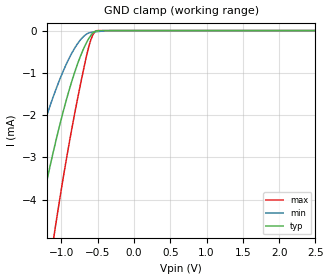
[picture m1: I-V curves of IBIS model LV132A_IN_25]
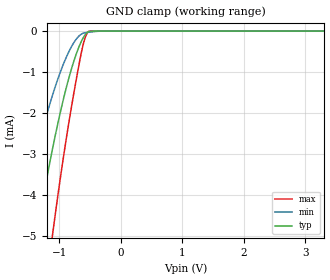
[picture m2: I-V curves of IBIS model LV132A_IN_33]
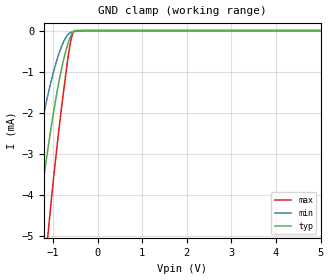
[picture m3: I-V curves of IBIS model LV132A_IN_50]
| TEXAS INSTRUMENTS INCORPORATED
| Standard Linear and Logic Group
| IBIS Model of SN74LV132A
| QUADRUPLE POSITIVE-NAND GATES WITH SCHMITT-TRIGGER INPUTS
| This file contains package information for the following:
|  SOIC 14-pin (D) package as [Component] LV132A_D
|  SSOP 14-pin (DB) package as [Component] LV132A_DB
|  TVSOP 14-pin (DGV) package as [Component] LV132A_DGV
|  SOP 14-pin (NS) package as [Component] LV132A_NS
|  TSSOP 14-pin (PW) package as [Component] LV132A_PW
| This device can be powered at the following Vccs:
|  2.5 volt Vcc
|  3.3 volt Vcc
|  5 volt Vcc
| This file provides unique models under the [Model Selector] for each Vcc.
| For operation at a specific Vcc, select the appropriate model after each
| [Model Selector] keyword.
[IBIS Ver]   3.2
[Comment char]  |_char
[File Name]   sn74lv132a.ibs
[File Rev]   1.1 | h_die
[Date]   February 26, 2004
[Source]   Data created from TI-SPICE simulations at TI-SLL.
[Notes]   The following is an IBIS list for the LV132A.
   Please contact sllibis@ti.com with questions and
   comments concerning SLL IBIS models.
   This IBIS model is created from a BA (back annotated netlist)
   - FILE REV HISTORY
   - 1.1 Release IBIS file on 02/26/04
   - Power clamp data deleted as there is no power-clamp diode.
[Disclaimer] Property of Texas Instruments Incorporated.  Unauthorized
   reproduction and/or distribution is strictly prohibited.
   This product is protected under copyright law.
   Created  2003, (C) Copyright  2003, Texas Instruments
   Incorporated, All Rights Reserved
   UNLESS THERE IS A SIGNED, WRITTEN AGREEMENT TO THE
   CONTRARY, TEXAS INSTRUMENTS (TI) IS PROVIDING THE IBIS
   MODELS  AND WITHOUT ANY WARRANTY, EXPRESSED OR
   IMPLIED.  TI assumes no liability for:
   1) the accuracy of the IBIS models provided to your
   company;
   2) the proper functioning of these IBIS Models in your
   design or for any resulting applications; or
   3) infringement of patents, copyrights or intellectual
   property rights resulting from your use of these IBIS
   models.
   TI provides IBIS Models as a service to our customers.
   You and your company shall not distribute, sell or give
   these models to anyone else without prior written
   permission from TI.
   TI reserves the right to make changes to our products or
   to discontinue any semiconductor product or service
   without notice, and advises our customers to obtain the
   latest version of relevant information to verify, before
   placing orders, that the information being relied on is
   current.
   Please be aware that your receipt and use of the IBIS
   information provided shall serve as acceptance of these
   terms and conditions.  If you do not accept these terms,
   you should return or destroy the IBIS models and any
   other accompanying information immediately.
| Component LV132A_D 14-pin SOIC
[Component]   LV132A_D
[Manufacturer]   Texas Instruments, Inc.
[Package]
|   typ   min   max
R_pkg   3.100e-02   2.800e-02   3.400e-02
L_pkg   3.109e-09   2.462e-09   3.889e-09
C_pkg   4.730e-13   3.630e-13   6.280e-13
[Pin]   signal_name   model_name   R_pin   L_pin   C_pin
1   1A   LV132A_IN   3.300e-02   3.854e-09   6.220e-13
2   1B   LV132A_IN   3.200e-02   3.188e-09   4.730e-13
3   1Y   LV132A_OUT   2.800e-02   2.462e-09   3.770e-13
4   2A   LV132A_IN   3.100e-02   2.596e-09   3.630e-13
5   2B   LV132A_IN   2.800e-02   2.521e-09   3.720e-13
6   2Y   LV132A_OUT   3.400e-02   3.250e-09   4.760e-13
7   GND   GND   3.400e-02   3.889e-09   6.280e-13
8   3Y   LV132A_OUT   3.400e-02   3.889e-09   6.280e-13
9   3A   LV132A_IN   3.400e-02   3.250e-09   4.760e-13
10   3B   LV132A_IN   2.800e-02   2.521e-09   3.720e-13
11   4Y   LV132A_OUT   3.100e-02   2.596e-09   3.640e-13
12   4A   LV132A_IN   2.800e-02   2.462e-09   3.770e-13
13   4B   LV132A_IN   3.200e-02   3.188e-09   4.730e-13
14   VCC   POWER   3.300e-02   3.854e-09   6.220e-13
| Component LV132A_DB 14-pin SSOP
[Component]   LV132A_DB
[Manufacturer]   Texas Instruments, Inc.
[Package]
|   typ   min   max
R_pkg   4.400e-02   4.100e-02   4.600e-02
L_pkg   3.551e-09   3.258e-09   3.927e-09
C_pkg   4.020e-13   3.600e-13   4.210e-13
[Pin]   signal_name   model_name   R_pin   L_pin   C_pin
1   1A   LV132A_IN   4.600e-02   3.927e-09   4.080e-13
2   1B   LV132A_IN   4.400e-02   3.587e-09   4.210e-13
3   1Y   LV132A_OUT   4.100e-02   3.289e-09   3.980e-13
4   2A   LV132A_IN   4.200e-02   3.258e-09   3.600e-13
5   2B   LV132A_IN   4.100e-02   3.286e-09   4.030e-13
6   2Y   LV132A_OUT   4.400e-02   3.586e-09   4.210e-13
7   GND   GND   4.600e-02   3.927e-09   4.080e-13
8   3Y   LV132A_OUT   4.600e-02   3.927e-09   4.080e-13
9   3A   LV132A_IN   4.400e-02   3.586e-09   4.210e-13
10   3B   LV132A_IN   4.100e-02   3.286e-09   4.030e-13
11   4Y   LV132A_OUT   4.300e-02   3.258e-09   3.600e-13
12   4A   LV132A_IN   4.100e-02   3.289e-09   3.980e-13
13   4B   LV132A_IN   4.400e-02   3.587e-09   4.210e-13
14   VCC   POWER   4.600e-02   3.927e-09   4.080e-13
| Component LV132A_DGV 14-pin TVSOP
[Component]   LV132A_DGV
[Manufacturer]   Texas Instruments, Inc.
[Package]
|   typ   min   max
R_pkg   3.500e-02   2.000e-02   4.500e-02
L_pkg   2.499e-09   2.077e-09   2.966e-09
C_pkg   3.610e-13   3.050e-13   4.160e-13
[Pin]   signal_name   model_name   R_pin   L_pin   C_pin
1   1A   LV132A_IN   2.700e-02   2.717e-09   3.730e-13
2   1B   LV132A_IN   3.700e-02   2.434e-09   3.980e-13
3   1Y   LV132A_OUT   3.400e-02   2.200e-09   3.160e-13
4   2A   LV132A_IN   2.000e-02   2.077e-09   3.090e-13
5   2B   LV132A_IN   3.000e-02   2.147e-09   3.050e-13
6   2Y   LV132A_OUT   4.200e-02   2.580e-09   4.080e-13
7   GND   GND   3.900e-02   2.921e-09   3.850e-13
8   3Y   LV132A_OUT   3.300e-02   2.841e-09   3.800e-13
9   3A   LV132A_IN   4.200e-02   2.611e-09   4.100e-13
10   3B   LV132A_IN   3.800e-02   2.331e-09   3.290e-13
11   4Y   LV132A_OUT   2.600e-02   2.223e-09   3.190e-13
12   4A   LV132A_IN   3.400e-02   2.259e-09   3.130e-13
13   4B   LV132A_IN   4.500e-02   2.681e-09   4.160e-13
14   VCC   POWER   4.200e-02   2.966e-09   3.860e-13
| Component LV132A_NS 14-pin SOP
[Component]   LV132A_NS
[Manufacturer]   Texas Instruments, Inc.
[Package]
|   typ   min   max
R_pkg   4.500e-02   3.900e-02   5.400e-02
L_pkg   3.796e-09   2.561e-09   4.952e-09
C_pkg   5.280e-13   2.880e-13   7.100e-13
[Pin]   signal_name   model_name   R_pin   L_pin   C_pin
1   1A   LV132A_IN   4.700e-02   4.867e-09   7.060e-13
2   1B   LV132A_IN   5.100e-02   4.083e-09   5.920e-13
3   1Y   LV132A_OUT   4.100e-02   2.915e-09   3.760e-13
4   2A   LV132A_IN   3.900e-02   2.561e-09   2.880e-13
5   2B   LV132A_IN   4.100e-02   3.101e-09   4.300e-13
6   2Y   LV132A_OUT   4.700e-02   4.047e-09   5.890e-13
7   GND   GND   5.100e-02   4.909e-09   7.000e-13
8   3Y   LV132A_OUT   4.500e-02   4.784e-09   6.940e-13
9   3A   LV132A_IN   5.400e-02   4.176e-09   5.970e-13
10   3B   LV132A_IN   3.900e-02   3.287e-09   4.490e-13
11   4Y   LV132A_OUT   3.900e-02   2.586e-09   2.940e-13
12   4A   LV132A_IN   4.000e-02   2.802e-09   3.710e-13
13   4B   LV132A_IN   4.900e-02   4.080e-09   5.930e-13
14   VCC   POWER   5.200e-02   4.952e-09   7.100e-13
| Component LV132A_PW 14-pin TSSOP
[Component]   LV132A_PW
[Manufacturer]   Texas Instruments, Inc.
[Package]
|   typ   min   max
R_pkg   3.200e-02   2.900e-02   3.500e-02
L_pkg   2.378e-09   2.170e-09   2.680e-09
C_pkg   3.140e-13   2.700e-13   3.350e-13
[Pin]   signal_name   model_name   R_pin   L_pin   C_pin
1   1A   LV132A_IN   3.300e-02   2.618e-09   3.300e-13
2   1B   LV132A_IN   3.100e-02   2.313e-09   3.170e-13
3   1Y   LV132A_OUT   3.000e-02   2.310e-09   3.140e-13
4   2A   LV132A_IN   3.100e-02   2.173e-09   2.720e-13
5   2B   LV132A_IN   3.000e-02   2.204e-09   3.090e-13
6   2Y   LV132A_OUT   3.200e-02   2.315e-09   3.170e-13
7   GND   GND   3.500e-02   2.680e-09   3.350e-13
8   3Y   LV132A_OUT   3.300e-02   2.640e-09   3.330e-13
9   3A   LV132A_IN   3.400e-02   2.347e-09   3.190e-13
10   3B   LV132A_IN   2.900e-02   2.277e-09   3.130e-13
11   4Y   LV132A_OUT   3.100e-02   2.170e-09   2.700e-13
12   4A   LV132A_IN   3.100e-02   2.244e-09   3.110e-13
13   4B   LV132A_IN   3.300e-02   2.343e-09   3.210e-13
14   VCC   POWER   3.500e-02   2.657e-09   3.320e-13
| Model LV132A_IN
[Model Selector]   LV132A_IN
LV132A_IN_25   2.5 volt Vcc
LV132A_IN_33   3.3 volt Vcc
LV132A_IN_50   5 volt Vcc
| Model LV132A_OUT
[Model Selector]   LV132A_OUT
LV132A_OUT_25   2.5 volt Vcc
LV132A_OUT_33   3.3 volt Vcc
LV132A_OUT_50   5 volt Vcc
| Models and submodels in the file (6): LV132A_IN_25 (Input), LV132A_IN_33 (Input), LV132A_IN_50 (Input), LV132A_OUT_25 (Output), LV132A_OUT_33 (Output), LV132A_OUT_50 (Output)
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[Model]   LV132A_IN_25
Model_type  Input
Vinl = 0.69
Vinh = 1.89
| variable   typ   min   max
C_comp   1.18pF   0.75pF   1.38pF
[Temperature Range]   40   100   -40
| Ambient temperature   25   85   -40
[Voltage range]   2.5   2.3   2.7
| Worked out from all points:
|   GND clamp passes 1 mA (typ) near -0.82 V on its own axis
[GND Clamp]
| LV132A_IN_25
|   Voltage   I(typ)   I(min)   I(max)
-2.5V     -17.05mA   -11.36mA   -25.61mA
-1.66V    -7.706mA   -4.815mA   -12.15mA
-1.63V    -7.409mA   -4.61mA    -11.71mA
-1.335V   -4.669mA   -2.746mA   -7.68mA
-1.095V   -2.745mA   -1.481mA   -4.777mA
-975mV    -1.913mA   -958.1uA   -3.482mA
-855mV    -1.189mA   -528.2uA   -2.306mA
-750mV    -661.2uA   -245.3uA   -1.378mA
-645mV    -255.5uA   -74.6uA    -531.1uA
-575mV    -74.68uA   -38.44uA   -133.8uA
-515mV    -7.128uA   -26.16uA   -2.186uA
2.5V      10.21pA    144.7pA    7.51pA
[Model]   LV132A_IN_33
Model_type  Input
Vinl = 0.9
Vinh = 2.52
| variable   typ   min   max
C_comp   1.19pF   0.74pF   1.37pF
[Temperature Range]   40   100   -40
| Ambient temperature   25   85   -40
[Voltage range]   3.3   3   3.6
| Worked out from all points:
|   GND clamp passes 1 mA (typ) near -0.82 V on its own axis
[GND Clamp]
| LV132A_IN_33
|   Voltage   I(typ)   I(min)   I(max)
-3.3V     -27.15mA   -18.54mA   -40.03mA
-1.675V   -7.856mA   -4.918mA   -12.36mA
-1.365V   -4.931mA   -2.922mA   -8.068mA
-1.225V   -3.748mA   -2.134mA   -6.301mA
-1.105V   -2.818mA   -1.528mA   -4.89mA
-965mV    -1.849mA   -918.5uA   -3.379mA
-850mV    -1.162mA   -512.6uA   -2.26mA
-725mV    -552.3uA   -193.2uA   -1.168mA
-625mV    -195.3uA   -58.14uA   -394.4uA
-570mV    -65.36uA   -37.36uA   -114.8uA
-510mV    -6.292uA   -25.2uA    -1.454uA
3.3V      13.4pA     149.4pA    9.907pA
[Model]   LV132A_IN_50
Model_type  Input
Vinl = 1.35
Vinh = 3.85
| variable   typ   min   max
C_comp   1.19pF   0.75pF   1.35pF
[Temperature Range]   40   100   -40
| Ambient temperature   25   85   -40
[Voltage range]   5   4.5   5.5
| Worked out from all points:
|   GND clamp passes 1 mA (typ) near -0.82 V on its own axis
[GND Clamp]
| LV132A_IN_50
|   Voltage   I(typ)   I(min)   I(max)
-5V       -50.6mA    -35.31mA   -73.31mA
-1.695V   -8.057mA   -5.057mA   -12.66mA
-1.64V    -7.507mA   -4.678mA   -11.86mA
-1.35V    -4.799mA   -2.834mA   -7.873mA
-1.11V    -2.855mA   -1.552mA   -4.946mA
-975mV    -1.913mA   -958.1uA   -3.482mA
-835mV    -1.08mA    -466.9uA   -2.123mA
-710mV    -490.5uA   -165.2uA   -1.044mA
-610mV    -154.3uA   -49.56uA   -303.2uA
-555mV    -40.93uA   -34.18uA   -66.31uA
-510mV    -6.292uA   -25.2uA    -1.454uA
5V        20.25pA    158.4pA    15.01pA
